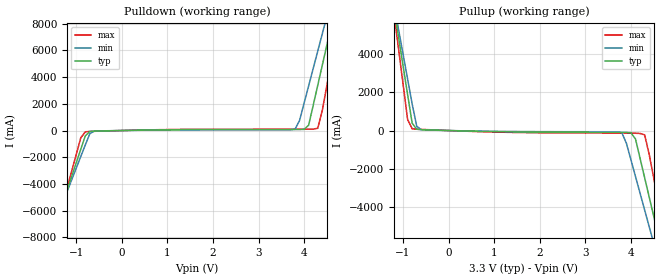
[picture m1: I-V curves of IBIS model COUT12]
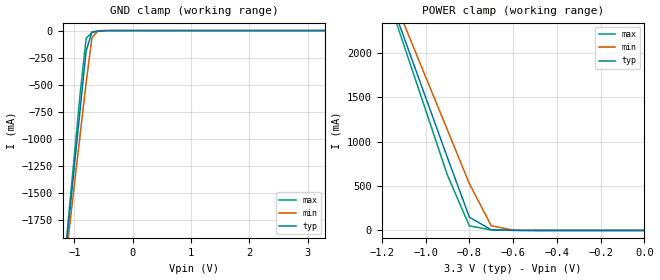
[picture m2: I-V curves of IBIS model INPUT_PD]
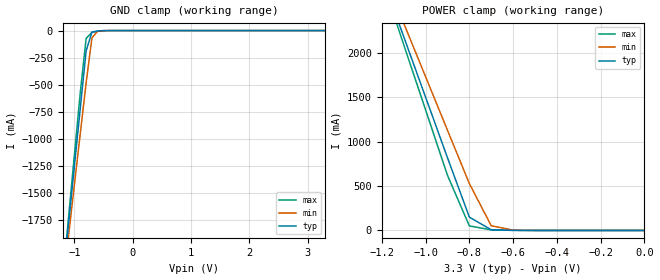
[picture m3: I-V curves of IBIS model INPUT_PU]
|   This file is an IBIS representation of the   |
|   Integrated Device Technology,Inc.   |
|   ICS840002i-01   |
|   LVCMOS/LVTTL Frequency Synthesizer   |
[IBIS Ver]   4.0
[File name]   840002i-01_3v3.ibs
[File Rev]   1.0
[Date]   Dec 11 2007 | Last Modified
|   Dec 11 2007 | Generated
[Source] Originated at Integrated Device Technology,Inc
[Disclaimer]
IDT hereby grants the user of this IBIS model a non-exclusive,
nontransferable license to use this IBIS model under the following terms.
Before using this IBIS model, the user should read this license.
If the user does not accept these terms,  the IBIS model should be
returned to IDT within 30 days.
   The user is granted this license only to use the IBIS model and
is not granted rights to sell, load, rent, lease or license the IBIS
model in whole or in part, or in modified form to anyone other than
user. User may modify the IBIS model to suit its specific
applications but rights to derivative works and such modifications
shall belong to IDT.
   This IBIS model is provided on an "AS IS" basis and IDT makes
absolutely no warranty with respect to the information contained
herein. ICS DISCLAIMS AND CUSTOMER WAIVES ALL WARRANTIES, EXPRESS
OR IMPLIED, INCLUDING WARRANTIES OF MERCHANTABILITY OR FITNESS FOR
A PARTICULAR PURPOSE. The entire risk as to quality and performance
is with the Customer. ACCORDINGLY, IN NO EVENT SHALL THE COMPANY BE
LIABLE FOR ANY DAMAGES, WHETHER IN CONTRACT OR TORT,INCLUDING ANY
LOST PROFITS OR OTHER INCIDENTAL, CONSEQUENTIAL, EXEMPLARY, OR
PUNITIVE DAMAGES ARISING OUT OF THE USE OR APPLICATION OF THE IBIS
model provided in this package. Further, IDT reserves the right to
make changes without notice to any product herein to improve
reliability, function, or design. IDT does not convey any license
under patent rights or any other intellectual property rights,
including those of third parties.
   IDT is not obligated to provide maintenance or support
for the licensed IBIS model.
[Copyright]   Copyright 2007 by Integrated Device Technology,Inc
[Component]   ICS840002AGI-01
[Manufacturer] Integrated Device Technology,Inc
[Package]
|   TSSOP16   typ   min   max
R_pkg   58.65m   52.5m   64.8m
L_pkg   1.902nH   1.443nH   2.361nH
C_pkg   0.315pF   0.254pF   0.375pF
[Pin] signal_name   model_name   R_pin   L_pin   C_pin
1   F_SEL0   INPUT_PU   64.8m   2.361n   0.375p
2   XTAL_SEL   INPUT_PD   60.7m   2.054n   0.335p
3   TEST_CLK   INPUT_PD   56.6m   1.749n   0.294p
4   OE   INPUT_PU   52.5m   1.443n   0.254p
5   MR   INPUT_PD   52.5m   1.443n   0.254p
6   nPLL_SEL   INPUT_PD   56.6m   1.749n   0.294p
7   VDDA   POWER   60.7m   2.054n   0.335p
8   VDD   POWER   64.8m   2.361n   0.375p
|9   XTAL_OUT   64.8m   2.361n   0.375p
|10  XTAL_IN   60.7m   2.054n   0.335p
11   VDDO   POWER   56.6m   1.749n   0.294p
12   Q1   COUT12   52.5m   1.443n   0.254p
13   Q0   COUT12   52.5m   1.443n   0.254p
14   GND   GND   56.6m   1.749n   0.294p
15   GND   GND   60.7m   2.054n   0.335p
16   FSEL1   INPUT_PU   64.8m   2.361n   0.375p
| Models and submodels in the file (3): COUT12 (Output), INPUT_PD (Input), INPUT_PU (Input)
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[Model]   COUT12
Model_type   Output
Polarity   Non-Inverting
Vmeas = 1.65
Rref = 50
Cref = 0
Vref = 1.65
|   typ   min   max
C_comp   2pF   1.5pF   2.5pF
|   typ   min   max
[Voltage range]  3.3V   3.15V   3.45V
|   typ   min   max
[Temperature Range]   27.0   -40   85
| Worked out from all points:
|   slope of the pulldown table from 0 to 0.495 V, typ, clamps not added: 15.4 ohm
|   slope of the pullup table from 0 to 0.495 V, typ, clamps not added: 15.2 ohm
[pulldown]
|Voltage   I (typ)   I (min)   I (max)
-3.3V     -25.76A    -22.97A    -30.46A
-1.5V     -7.499A    -7.2A      -8.039A
-900mV    -1.412A    -1.95A     -555.6mA
-800mV    -399.2mA   -1.076A    -95.23mA
-600mV    -44.85mA   -44.17mA   -58.2mA
3.8V      74.94mA    98.59mA    96.98mA
4.1V      400.7mA    3.343A     99.24mA
4.3V      3.388A     5.943A     169.6mA
4.4V      4.894A     7.244A     1.513A
4.6V      7.909A     9.846A     5.22A
4.8V      10.93A     12.45A     8.931A
6.6V      38.21A     35.99A     42.48A
[pullup]
|Voltage   I (typ)   I (min)   I (max)
-3.3V     38.17A     34.02A     45.19A
-1.2V     6.403A     6.598A     6.145A
-1.1V     4.892A     5.294A     4.286A
-900mV    1.87A      2.687A     569.6mA
-800mV    383.2mA    1.384A     89.62mA
-600mV    45.84mA    44mA       59.23mA
3.8V      -96.26mA   -112.7mA   -131.6mA
4.1V      -444.3mA   -2.407A    -142.4mA
4.3V      -2.464A    -4.151A    -227.1mA
4.6V      -5.499A    -6.77A     -3.731A
4.8V      -7.524A    -8.517A    -6.22A
6.6V      -25.76A    -24.26A    -28.62A
[Ramp]
|   typ   min   max
dV/dt_r   1.98/0.6n   1.98/0.80n   1.98/0.4n
dV/dt_f   1.98/0.6n   1.98/0.80n   1.98/0.4n
[Model]   INPUT_PD
Model_type   Input
Polarity   Non-Inverting
Vinl = 1.4V
Vinh = 1.85V
|   typ   min   max
C_comp   2pF   1.5pF   2.5pF
|   typ   min   max
[Voltage range]  3.3V   3.15V   3.45V
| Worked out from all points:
|   GND clamp passes 1 mA (typ) near -0.51 V on its own axis
|   POWER clamp passes 1 mA (typ) near -0.60 V on its own axis
[GND_clamp]
|Voltage I(typ)   I(min)   I(max)
-3.3V     -13.52A    -12.28A    -14.38A
-1.2V     -2.314A    -2.362A    -2.296A
-1.1V     -1.782A    -1.891A    -1.721A
-1V       -1.25A     -1.422A    -1.146A
-900mV    -718.5mA   -952.6mA   -572.1mA
-800mV    -188.2mA   -484.5mA   -72.95mA
-700mV    -13.66mA   -66.68mA   -15.82mA
-600mV    -3.044mA   -4.415mA   -6.968mA
-500mV    -658.9uA   -400.5uA   -2.169mA
3.3V      64.58uA    64.62uA    64.6uA
[POWER_clamp]
|Voltage   I(typ)   I(min)   I(max)
-3.3V     17.27A     15.67A     18.38A
-1.2V     2.866A     2.938A     2.832A
-1.1V     2.183A     2.334A     2.094A
-1V       1.501A     1.732A     1.358A
-900mV    819.8mA    1.13A      621.9mA
-800mV    150.3mA    528.4mA    51.58mA
-700mV    7.809mA    53.45mA    6.607mA
-600mV    968.4uA    3.161mA    1.955mA
0V        64.58uA    61.35uA    67.83uA
[Model]   INPUT_PU
Model_type   Input
Polarity   Non-Inverting
Vinl = 1.4V
Vinh = 1.85V
|   typ   min   max
C_comp   2pF   1.5pF   2.5pF
|   typ   min   max
[Voltage range]  3.3V   3.15V   3.45V
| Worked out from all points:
|   GND clamp passes 1 mA (typ) near -0.51 V on its own axis
|   POWER clamp passes 1 mA (typ) near -0.60 V on its own axis
[GND_clamp]
|Voltage   I(typ)   I(min)   I(max)
-3.3V     -13.52A    -12.28A    -14.38A
-1.2V     -2.314A    -2.362A    -2.296A
-1.1V     -1.782A    -1.891A    -1.721A
-1V       -1.25A     -1.422A    -1.146A
-900mV    -718.6mA   -952.7mA   -572.2mA
-800mV    -188.2mA   -484.6mA   -73.02mA
-700mV    -13.72mA   -66.74mA   -15.89mA
-600mV    -3.109mA   -4.477mA   -7.036mA
-500mV    -723.5uA   -462.1uA   -2.236mA
3.3V      3.748nA    2.972uA    -2.918uA
[POWER_clamp]
|Voltage   I(typ)   I(min)   I(max)
-3.3V     17.27A     15.67A     18.38A
-1.2V     2.866A     2.938A     2.832A
-1.1V     2.183A     2.334A     2.094A
-1V       1.501A     1.732A     1.358A
-900mV    819.7mA    1.129A     621.8mA
-800mV    150.2mA    528.4mA    51.51mA
-700mV    7.744mA    53.39mA    6.54mA
-600mV    903.9uA    3.099mA    1.887mA
0V        3.748nA    2.31nA     19.96nA
